| IBIS file generated by GenIBIS.pl Version 3.20
|   dm8168_pg2x
[IBIS ver]   4.1
[File name]   sprm568.ibs
[File Rev]   2.2
[Date]   Mon May 21, 2012, 13:39:56
[Source]   Data created at Texas Instruments
[Notes]   Checked with ibisckr
   16 warnings can be waived
   Some pins may contain selectors which are not valid options
   for that particular pin.
   Please refer to the device datasheet for information on picking
   the correct selector model, which depends on various software
   register configurations.
   Some pins are modeled as IO or tri-state for output mode.
[Disclaimer] Please be aware that in the absence of a written agreement,
   Texas Instruments (TI) assumes no liability for: 1) the
   accuracy of the IBIS models provided to your company, 2) the
   proper functioning of these IBIS models in your design or for
   any resulting applications, or, 3) infringement of patents,
   copyrights, or intellectual property rights resulting from
   your use of these IBIS models. TI provides IBIS models as a
   service to our customers and therefore reserves the right to
   limit distribution of the IBIS models.
[Copyright]   Property of Texas Instruments Incorporated. Unauthorised
   reproduction and/or distribution is strictly prohibited. This
   product is protected under copyright law and trade secret law
   as an unpublished work. Created 2010,(C) Copyright 2010,
   Texas Instruments Incorporated., All Rights Reserved. These
   commodities are under the U.S. Government distribution license
   control.As such,they are not to be re-exported without the
   prior approval of the U.S. Department of Commerce.
|   Component dm8168_pg2x
[Component]   dm8168_pg2x
[Manufacturer]   Texas Instruments.
| Source IO level model revisions
|Model   Revision   Date
|BSHTLTCSCDVGPBFZ   1.4   Jan 5, 2011
|IHHV33GP18   1.0   Feb 18, 2010
|BSHTLTCSCDDVGPBFZ   1.4   Jan 5, 2011
|BI2C33GFZP18   1.0   Feb 18, 2010
|BC3340CGHYPBFBP18   1.0   Feb 18, 2010
|BC3340DGHYPBFBP18   1.0   Feb 18, 2010
|IQ33GHYPBFBP18   1.0   Feb 18, 2010
[Package]
|   typ   min   max
R_pkg   1083.455m   49.41m   2117.50m
L_pkg   3.26nH   0.72nH   5.80nH
C_pkg   1.675pF   0.63pF   2.72pF
[Pin]   signal_name   model_name   R_pin   L_pin   C_pin
H37   CLKIN32   Selector_5   1309.20m   3.65nH   1.83pF
F1   CLKOUT   Selector_5   1491.00m   3.78nH   1.94pF
F18   DDR[0]_CS[1]N   Selector_6   1308.20m   3.34nH   1.73pF
G4   DDR[0]_D[3]   Selector_4   1490.40m   3.74nH   2.07pF
G34   DDR[1]_D[3]   Selector_4   1489.80m   3.78nH   2.08pF
C18   DDR[0]_CKE   Selector_6   1358.20m   3.54nH   1.63pF
N14   DDR[0]_A[8]   Selector_6   1151.50m   3.06nH   1.57pF
B2   DDR[0]_D[5]   Selector_4   1489.90m   3.72nH   2.04pF
A31   DDR[1]_D[17]   Selector_4   1477.60m   3.79nH   1.89pF
C29   DDR[1]_D[31]   Selector_4   1476.80m   3.76nH   1.94pF
F29   DDR[1]_D[22]   Selector_4   1441.70m   3.68nH   1.89pF
C37   DDR[1]_D[7]   Selector_4   1538.40m   3.97nH   2.11pF
D6   DDR[0]_D[11]   Selector_4   1736.00m   3.98nH   2.27pF
A7   DDR[0]_D[17]   Selector_4   1476.50m   3.78nH   1.93pF
J25   DDR[1]_A[5]   Selector_6   1309.60m   3.41nH   1.73pF
D32   DDR[1]_D[11]   Selector_4   1733.00m   4.16nH   2.21pF
B32   DDR[1]_D[13]   Selector_4   1708.80m   4.35nH   2.32pF
H25   DDR[1]_A[4]   Selector_6   1241.80m   3.15nH   1.69pF
B14   DDR[0]_BA[1]   Selector_6   1319.50m   3.63nH   1.86pF
C25   DDR[1]_CASN   Selector_6   1319.50m   3.60nH   1.85pF
B37   DDR[1]_D[0]   Selector_4   1469.70m   3.83nH   2.00pF
A32   DDR[1]_VTP   NC
B17   DDR[0]_CS[0]N   Selector_6   1349.40m   3.49nH   1.72pF
C8   DDR[0]_D[16]   Selector_4   1423.40m   3.34nH   1.91pF
A26   DDR[1]_CLK[0]N   Selector_6   1408.90m   3.58nH   1.67pF
B28   DDR[1]_D[26]   Selector_4   1457.10m   3.72nH   1.90pF
N21   DDR[1]_A[1]   Selector_6   1193.70m   3.19nH   1.60pF
B30   DDR[1]_DQS[2]   Selector_1   1543.40m   3.74nH   1.70pF
C14   DDR[0]_A[10]   Selector_6   1298.30m   3.51nH   1.79pF
F9   DDR[0]_D[22]   Selector_4   1439.50m   3.61nH   1.90pF
A9   DDR[0]_DQS[3]N   Selector_1   1585.40m   3.85nH   1.84pF
B7   DDR[0]_D[19]   Selector_4   1383.00m   3.34nH   1.95pF
A3   DDR[0]_D[14]   Selector_4   1766.10m   4.41nH   2.34pF
B1   DDR[0]_D[0]   Selector_4   1470.70m   3.76nH   2.13pF
A15   DDR[0]_CLK[1]   Selector_6   1409.10m   3.47nH   1.71pF
H13   DDR[0]_A[4]   Selector_6   1256.10m   3.18nH   1.74pF
D7   DDR[0]_D[9]   Selector_4   1744.10m   4.10nH   2.16pF
C24   DDR[1]_A[10]   Selector_6   1281.10m   3.40nH   1.81pF
D36   DDR[1]_D[4]   Selector_4   1532.20m   3.94nH   2.16pF
A35   DDR[1]_D[14]   Selector_4   1761.50m   4.48nH   2.31pF
F30   DDR[1]_D[20]   Selector_4   1426.70m   3.75nH   1.94pF
A4   DDR[0]_DQS[1]N   Selector_1   1881.10m   4.39nH   2.13pF
D31   DDR[1]_D[9]   Selector_4   1747.90m   4.19nH   2.19pF
A6   DDR[0]_VTP   NC
E18   DDR[0]_ODT[0]   Selector_6   1256.70m   3.57nH   1.67pF
B21   DDR[1]_CS[0]N   Selector_6   1338.00m   3.57nH   1.74pF
D20   DDR[1]_RSTN   Selector_6   1302.90m   3.49nH   1.67pF
N22   DDR[1]_A[12]   Selector_6   1129.60m   3.36nH   1.44pF
E2   DDR[0]_D[2]   Selector_4   1529.70m   3.83nH   2.00pF
A12   DDR[0]_CLK[0]N   Selector_6   1403.00m   3.48nH   1.71pF
G28   DDR[1]_D[28]   Selector_4   1477.50m   3.63nH   2.05pF
E29   DDR[1]_D[24]   NC
D30   DDR[1]_D[21]   Selector_4   1394.40m   3.59nH   1.98pF
C9   DDR[0]_D[31]   Selector_4   1469.70m   3.53nH   1.82pF
K13   DDR[0]_A[9]   Selector_6   1252.40m   3.22nH   1.70pF
G29   DDR[1]_DQM[2]   Selector_6   1449.00m   3.60nH   1.92pF
B3   DDR[0]_D[15]   Selector_4   1746.20m   4.07nH   2.26pF
A24   DDR[1]_A[7]   Selector_6   1317.50m   3.61nH   1.88pF
F36   DDR[1]_D[1]   Selector_4   1516.50m   3.72nH   2.10pF
B26   DDR[1]_CLK[0]   Selector_6   1421.50m   3.73nH   1.56pF
E7   DDR[0]_D[23]   NC
G13   DDR[0]_A[3]   Selector_6   1313.50m   3.47nH   1.69pF
B33   DDR[1]_DQM[1]   Selector_6   1739.30m   4.30nH   2.28pF
B35   DDR[1]_D[15]   Selector_4   1754.70m   4.28nH   2.24pF
G9   DDR[0]_DQM[2]   Selector_6   1448.90m   3.58nH   1.95pF
A30   DDR[1]_DQS[2]N   Selector_1   1544.90m   3.83nH   1.76pF
B10   DDR[0]_D[26]   Selector_4   1460.70m   3.63nH   1.97pF
E25   DDR[1]_WEN   Selector_6   1267.60m   3.39nH   1.80pF
F20   DDR[1]_CS[1]N   Selector_6   1298.80m   3.39nH   1.72pF
D18   DDR[0]_RSTN   Selector_6   1315.90m   3.41nH   1.71pF
F8   DDR[0]_D[20]   Selector_4   1427.80m   3.64nH   1.98pF
A34   DDR[1]_DQS[1]N   Selector_1   1885.10m   4.38nH   2.14pF
E36   DDR[1]_D[2]   Selector_4   1529.70m   3.92nH   2.08pF
A29   DDR[1]_DQS[3]N   Selector_1   1598.60m   3.83nH   1.94pF
G10   DDR[0]_D[28]   Selector_4   1486.50m   3.61nH   2.07pF
E35   DDR[1]_DQS[0]N   Selector_1   1600.60m   3.84nH   1.86pF
A13   DDR[0]_A[0]   Selector_6   1265.50m   3.65nH   1.74pF
E8   DDR[0]_D[27]   Selector_4   1430.00m   3.59nH   1.99pF
B9   DDR[0]_DQS[3]   Selector_1   1600.40m   3.82nH   1.84pF
F25   DDR[1]_BA[0]   Selector_6   1249.40m   3.21nH   1.71pF
E31   DDR[1]_D[23]   Selector_4   1404.30m   3.60nH   2.03pF
F13   DDR[0]_BA[0]   Selector_6   1260.70m   3.24nH   1.75pF
B11   DDR[0]_D[25]   Selector_4   1487.80m   3.56nH   1.92pF
J13   DDR[0]_A[5]   Selector_6   1333.50m   3.39nH   1.68pF
C13   DDR[0]_CASN   Selector_6   1332.10m   3.61nH   1.86pF
B25   DDR[1]_A[11]   Selector_6   1335.80m   3.85nH   1.84pF
J11   DDR[0]_D[30]   Selector_4   1504.00m   3.69nH   1.90pF
A8   DDR[0]_DQS[2]N   Selector_1   1538.30m   3.73nH   1.90pF
D8   DDR[0]_D[21]   Selector_4   1394.50m   3.33nH   2.05pF
A33   DDR[1]_D[12]   Selector_4   1736.90m   4.33nH   2.28pF
C11   DDR[0]_D[29]   Selector_4   1449.60m   3.76nH   1.97pF
A5   DDR[0]_D[12]   Selector_4   1740.90m   4.25nH   2.37pF
D15   DDR[0]_A[2]   Selector_6   1293.60m   3.44nH   1.80pF
B4   DDR[0]_DQS[1]   Selector_1   1878.40m   4.27nH   2.13pF
C30   DDR[1]_D[16]   Selector_4   1420.60m   3.50nH   2.00pF
B29   DDR[1]_DQS[3]   Selector_1   1607.10m   4.02nH   1.86pF
H10   DDR[0]_D[18]   Selector_4   1427.20m   3.35nH   2.06pF
E13   DDR[0]_WEN   Selector_6   1287.90m   3.35nH   1.78pF
D17   DDR[0]_A[14]   Selector_6   1253.70m   3.19nH   1.81pF
A25   DDR[1]_A[0]   Selector_6   1266.80m   3.73nH   1.79pF
C32   DDR[1]_D[10]   Selector_4   1784.80m   4.48nH   2.18pF
B13   DDR[0]_A[11]   Selector_6   1352.50m   3.67nH   1.95pF
A14   DDR[0]_A[7]   NC
F2   DDR[0]_D[1]   Selector_4   1518.50m   3.74nH   2.08pF
B36   DDR[1]_D[5]   Selector_4   1496.60m   3.79nH   2.09pF
L13   DDR[0]_A[6]   Selector_6   1153.10m   3.02nH   1.61pF
H28   DDR[1]_D[18]   Selector_4   1427.50m   3.48nH   1.90pF
F35   DDR[1]_D[6]   Selector_4   1543.90m   3.99nH   2.08pF
N16   DDR[0]_A[12]   Selector_6   1122.70m   3.13nH   1.44pF
B34   DDR[1]_DQS[1]   Selector_1   1881.40m   4.41nH   2.08pF
C36   DDR[1]_DQM[0]   Selector_6   1526.50m   4.01nH   2.09pF
F34   DDR[1]_DQS[0]   Selector_1   1622.30m   3.89nH   1.76pF
L25   DDR[1]_A[6]   Selector_6   1146.20m   2.92nH   1.59pF
A23   DDR[1]_CLK[1]   Selector_6   1408.60m   3.54nH   1.77pF
A22   DDR[1]_ODT[1]   Selector_6   1360.60m   3.61nH   1.87pF
F4   DDR[0]_DQS[0]   Selector_1   1620.50m   3.95nH   1.97pF
D25   DDR[1]_RASN   Selector_6   1251.90m   3.31nH   1.80pF
D21   DDR[1]_A[14]   Selector_6   1262.30m   3.15nH   1.77pF
D29   DDR[1]_DQM[3]   Selector_6   1482.20m   3.81nH   2.01pF
B16   DDR[0]_A[13]   Selector_6   1270.10m   3.37nH   1.81pF
N15   DDR[0]_BA[2]   Selector_6   1133.30m   3.22nH   1.44pF
E30   DDR[1]_D[27]   Selector_4   1425.40m   3.68nH   2.08pF
B27   DDR[1]_D[25]   Selector_4   1494.60m   3.90nH   1.92pF
C20   DDR[1]_CKE   Selector_6   1327.50m   3.43nH   1.63pF
N24   DDR[1]_A[8]   Selector_6   1151.30m   3.03nH   1.54pF
B12   DDR[0]_CLK[0]   Selector_6   1415.20m   3.69nH   1.69pF
B6   DDR[0]_D[13]   Selector_4   1710.40m   4.12nH   2.18pF
N23   DDR[1]_BA[2]   Selector_6   1141.30m   3.31nH   1.43pF
F3   DDR[0]_D[6]   Selector_4   1543.60m   4.02nH   2.09pF
C27   DDR[1]_D[29]   Selector_4   1448.30m   3.80nH   2.01pF
E9   DDR[0]_D[24]   Selector_4   1434.50m   3.63nH   1.86pF
J27   DDR[1]_D[30]   Selector_4   1507.60m   3.72nH   2.06pF
E20   DDR[1]_ODT[0]   Selector_6   1246.60m   3.51nH   1.69pF
B24   DDR[1]_BA[1]   Selector_6   1300.70m   3.55nH   1.82pF
A16   DDR[0]_ODT[1]   Selector_6   1375.80m   3.74nH   1.86pF
D13   DDR[0]_RASN   Selector_6   1266.70m   3.18nH   1.82pF
D2   DDR[0]_D[4]   Selector_4   1531.00m   3.98nH   2.12pF
D23   DDR[1]_A[2]   Selector_6   1279.00m   3.38nH   1.87pF
D9   DDR[0]_DQM[3]   Selector_6   1479.60m   3.74nH   1.92pF
B15   DDR[0]_CLK[1]N   Selector_6   1400.90m   3.42nH   1.71pF
N17   DDR[0]_A[1]   Selector_6   1196.40m   3.20nH   1.58pF
G25   DDR[1]_A[3]   Selector_6   1301.50m   3.47nH   1.74pF
K25   DDR[1]_A[9]   Selector_6   1252.70m   3.22nH   1.71pF
B31   DDR[1]_D[19]   Selector_4   1383.90m   3.59nH   1.84pF
E3   DDR[0]_DQS[0]N   Selector_1   1601.30m   3.84nH   1.94pF
B5   DDR[0]_DQM[1]   Selector_6   1739.40m   4.39nH   2.24pF
C33   DDR[1]_D[8]   NC
B22   DDR[1]_A[13]   Selector_6   1250.70m   3.43nH   1.78pF
B8   DDR[0]_DQS[2]   Selector_1   1535.10m   3.81nH   1.76pF
C5   DDR[0]_D[8]   Selector_4   1688.70m   3.78nH   2.09pF
B23   DDR[1]_CLK[1]N   Selector_6   1400.10m   3.58nH   1.69pF
C6   DDR[0]_D[10]   Selector_4   1782.00m   4.37nH   2.22pF
C2   DDR[0]_DQM[0]   Selector_6   1527.40m   3.89nH   2.14pF
C1   DDR[0]_D[7]   NC
A19   DEV_MXI   NC
C19   DEV_MXO   NC
AU31   EMAC[1]_TXD[4]   Selector_2   1696.40m   4.60nH   2.24pF
AD35   EMAC[0]_RXD[3]   Selector_2   947.25m   2.61nH   1.46pF
AT31   EMAC[1]_TXD[5]   Selector_2   1489.10m   4.26nH   1.93pF
AU30   EMAC[1]_TXEN   Selector_2   1493.30m   4.07nH   2.01pF
AU36   EMAC[1]_RXD[2]   Selector_2   1943.20m   4.97nH   2.40pF
AE36   EMAC[0]_RXD[7]   Selector_2   1288.30m   3.53nH   1.68pF
AU33   EMAC[1]_GMTCLK   Selector_2   1708.70m   4.59nH   2.17pF
AG36   EMAC[0]_TXD[6]   Selector_2   1331.80m   3.61nH   1.78pF
AT37   EMAC[1]_RXCLK   Selector_2   1743.20m   4.77nH   2.32pF
AT35   EMAC[1]_RXD[1]   Selector_2   1674.40m   4.57nH   2.13pF
AB25   EMAC[0]_COL   Selector_2   226.60m   1.06nH   0.71pF
AF37   EMAC[0]_TXCLK   Selector_2   1350.00m   3.67nH   1.87pF
AG37   EMAC[0]_TXEN   Selector_2   1452.10m   3.88nH   1.95pF
AT34   EMAC[1]_RXD[3]   Selector_2   1793.70m   4.65nH   2.21pF
AG35   EMAC[0]_TXD[7]   Selector_2   1051.50m   2.91nH   1.59pF
AT30   EMAC[1]_TXCLK   Selector_2   1568.10m   4.28nH   2.08pF
AE37   EMAC[0]_RXCLK   Selector_2   1509.90m   3.89nH   2.04pF
AD25   EMAC[0]_RXD[5]   Selector_2   170.60m   1.01nH   0.78pF
AC35   EMAC[0]_RXD[4]   Selector_2   1124.40m   3.09nH   1.69pF
AR33   EMAC[1]_RXD[5]   Selector_2   1589.90m   4.08nH   2.09pF
AP30   EMAC[1]_TXD[6]   Selector_2   1528.60m   4.24nH   1.97pF
AF36   EMAC[0]_TXD[5]   Selector_2   1240.00m   3.21nH   1.63pF
AP31   EMAC[1]_TXD[0]   Selector_2   1401.40m   3.88nH   1.91pF
AU32   EMAC[1]_TXD[3]   Selector_2   1538.00m   4.30nH   2.17pF
AE35   EMAC[0]_RXDV   Selector_2   1056.10m   2.91nH   1.55pF
AC36   EMAC[0]_RXD[2]   Selector_2   1200.10m   3.19nH   1.70pF
AP32   EMAC[1]_RXD[7]   Selector_2   1347.40m   3.62nH   1.88pF
AR32   EMAC[1]_TXD[1]   Selector_2   1395.10m   3.95nH   1.95pF
AE32   EMAC[0]_TXD[1]   Selector_2   762.14m   2.22nH   1.20pF
AU35   EMAC[1]_RXD[4]   Selector_2   1865.90m   4.74nH   2.42pF
AG28   EMAC[0]_TXD[4]   Selector_2   564.85m   1.69nH   1.08pF
AD37   EMAC[0]_RXD[0]   Selector_2   1306.50m   3.47nH   1.77pF
AD36   EMAC[0]_RXD[1]   Selector_2   1427.60m   3.90nH   1.76pF
AN30   EMAC[1]_RXER   Selector_2   1352.10m   3.58nH   1.79pF
AE31   EMAC[0]_TXD[2]   Selector_2   828.93m   2.29nH   1.22pF
AC25   EMAC[0]_RXD[6]   Selector_2   92.81m   0.81nH   0.65pF
AC37   EMAC[0]_GMTCLK   Selector_2   1221.60m   3.13nH   1.69pF
AR30   EMAC[1]_COL   Selector_2   1353.40m   3.90nH   1.89pF
AE33   EMAC[0]_TXD[0]   Selector_2   986.48m   2.66nH   1.40pF
AN31   EMAC[1]_CRS   Selector_2   1339.00m   3.72nH   1.83pF
AT32   EMAC[1]_TXD[2]   Selector_2   1667.80m   4.59nH   2.05pF
AE30   EMAC[0]_TXD[3]   Selector_2   493.69m   1.61nH   1.01pF
AU34   EMAC[1]_RXD[6]   Selector_2   1858.20m   5.09nH   2.51pF
AT36   EMAC[1]_RXD[0]   Selector_2   1623.80m   4.40nH   2.14pF
AE34   EMAC[0]_RXER   Selector_2   916.91m   2.56nH   1.42pF
AM30   EMAC[1]_TXD[7]   Selector_2   1204.30m   3.33nH   1.65pF
AA25   EMAC[0]_CRS   Selector_2   100.59m   0.85nH   0.71pF
AT33   EMAC[1]_RXDV   Selector_2   1519.30m   4.11nH   2.10pF
J35   EMU0   Selector_2   1645.80m   4.47nH   2.22pF
L36   EMU1   Selector_2   1287.90m   3.82nH   1.76pF
L37   EMU2   Selector_2   1334.20m   3.65nH   1.85pF
M36   EMU3   Selector_2   1079.80m   3.03nH   1.65pF
M37   EMU4   Selector_2   1302.60m   3.45nH   1.77pF
K31   GP0[0]   Selector_5   795.97m   2.24nH   1.35pF
L29   GP0[1]   Selector_5   694.30m   2.11nH   1.26pF
G2   GP0[5]   Selector_5   1205.80m   3.58nH   1.79pF
H35   GP0[7]   Selector_5   1083.40m   3.13nH   1.75pF
H32   GP0[4]   Selector_5   1092.10m   2.82nH   1.67pF
G5   GP0[6]   Selector_5   1196.30m   3.27nH   1.74pF
J31   GP0[3]   Selector_5   1017.90m   2.83nH   1.55pF
H4   GP0[25]   Selector_5   1249.30m   3.40nH   1.66pF
AC5   GP0[20]   Selector_5   1270.00m   3.50nH   1.93pF
K30   GP0[2]   Selector_5   925.22m   2.65nH   1.41pF
J5   GP1[13]   Selector_5   1061.30m   3.17nH   1.63pF
J32   GP1[30]   Selector_5   1020.50m   2.79nH   1.56pF
J33   GP1[31]   Selector_5   1137.80m   3.33nH   1.68pF
AA2   GPMC_D[5]   Selector_5   1118.40m   3.28nH   1.58pF
AE2   GPMC_A[5]   Selector_5   1495.60m   3.99nH   1.96pF
AE1   GPMC_A[4]   Selector_5   1377.50m   3.92nH   1.90pF
J1   GPMC_A[15]   Selector_5   1395.10m   3.87nH   1.92pF
AH7   GPMC_CS[0]N   Selector_5   1189.60m   3.37nH   1.71pF
AE6   GPMC_A[0]   Selector_5   1350.00m   3.73nH   2.00pF
AG9   GPMC_CS[3]N   Selector_5   1366.30m   3.85nH   2.05pF
AA3   GPMC_D[3]   Selector_5   1056.40m   2.99nH   1.56pF
W1   GPMC_D[11]   Selector_5   1141.60m   3.23nH   1.64pF
Y2   GPMC_D[7]   Selector_5   1171.80m   3.24nH   1.63pF
W2   GPMC_D[12]   Selector_5   966.20m   2.79nH   1.53pF
J2   GPMC_A[16]   Selector_5   1182.70m   3.29nH   1.76pF
Y1   GPMC_D[9]   Selector_5   1157.00m   3.26nH   1.75pF
AB2   GPMC_D[2]   Selector_5   1290.40m   3.51nH   1.73pF
AG2   GPMC_WEN   Selector_5   1545.10m   4.10nH   2.08pF
V3   GPMC_D[14]   Selector_5   1008.30m   2.79nH   1.47pF
W3   GPMC_D[10]   Selector_5   1112.50m   3.04nH   1.53pF
Y10   GPMC_D[6]   Selector_5   352.48m   1.25nH   0.89pF
AE3   GPMC_A[3]   Selector_5   1358.60m   3.79nH   1.85pF
V10   GPMC_D[13]   Selector_5   184.75m   0.89nH   0.73pF
AC1   GPMC_D[0]   Selector_5   1233.50m   3.39nH   1.85pF
V1   GPMC_CLK   Selector_5   1272.40m   3.48nH   1.79pF
K8   GPMC_A[27]   Selector_5   879.20m   2.55nH   1.43pF
J3   GPMC_A[24]   Selector_5   1308.40m   3.54nH   1.75pF
K2   GPMC_A[22]   Selector_5   1115.70m   3.16nH   1.71pF
AD8   GPMC_A[6]   Selector_5   1530.30m   4.11nH   2.05pF
AC2   GPMC_A[11]   Selector_5   1362.40m   3.66nH   1.85pF
AE4   GPMC_A[2]   Selector_5   1235.40m   3.43nH   1.67pF
AH2   GPMC_CS[2]N   Selector_5   1411.50m   3.83nH   2.11pF
AD3   GPMC_A[7]   Selector_5   1196.70m   3.32nH   1.73pF
Y3   GPMC_D[4]   Selector_5   1143.00m   3.16nH   1.62pF
J6   GPMC_A[26]   Selector_5   1225.70m   3.47nH   1.74pF
AD4   GPMC_A[8]   Selector_5   1152.80m   3.26nH   1.73pF
H5   GPMC_A[14]   Selector_5   1173.60m   3.57nH   1.70pF
AD1   GPMC_A[10]   Selector_5   1395.90m   3.72nH   1.87pF
W4   GPMC_D[8]   Selector_5   980.65m   2.85nH   1.47pF
AE7   GPMC_DIR   Selector_5   1320.10m   3.72nH   1.87pF
H3   GPMC_A[21]   Selector_5   1193.00m   3.32nH   1.78pF
AE10   GPMC_ADVN_ALE   Selector_5   1720.10m   4.77nH   2.21pF
AD2   GPMC_A[9]   Selector_5   1429.00m   3.83nH   1.94pF
H2   GPMC_A[12]   Selector_5   1117.60m   3.22nH   1.57pF
J4   GPMC_A[23]   Selector_5   1051.60m   2.94nH   1.64pF
H6   GPMC_A[13]   Selector_5   1045.70m   3.38nH   1.56pF
AE11   GPMC_BE0N_CLE   Selector_5   532.49m   1.84nH   1.17pF
AE9   GPMC_WPN   Selector_5   1318.70m   3.47nH   1.88pF
AH1   GPMC_CS[1]N   Selector_5   1653.70m   4.70nH   2.01pF
AF1   GPMC_BE1N   Selector_5   1416.40m   3.85nH   2.00pF
AE8   GPMC_WAIT   Selector_5   1441.30m   4.00nH   1.90pF
J7   GPMC_A[25]   Selector_5   1173.20m   3.20nH   1.70pF
AE5   GPMC_A[1]   Selector_5   1097.80m   3.10nH   1.66pF
AF2   GPMC_OE_REN   Selector_5   1476.20m   3.88nH   1.94pF
V2   GPMC_D[15]   Selector_5   1141.50m   3.10nH   1.63pF
AA4   GPMC_D[1]   Selector_5   1051.20m   2.95nH   1.51pF
AG3   GPMC_CS[4]N   Selector_5   1297.50m   3.69nH   1.80pF
AG1   GPMC_CS[5]N   Selector_5   1663.40m   4.38nH   2.09pF
AE24   HDMI_HPDET   Selector_5   316.48m   1.39nH   0.87pF
AT26   HDMI_TMDSDP1   NC
AT25   HDMI_TMDSDP0   NC
AU24   HDMI_TMDSCLKN   NC
AP25   HDMI_CEC   Selector_5   1161.80m   3.19nH   1.63pF
AU25   HDMI_TMDSDN0   NC
AU26   HDMI_TMDSDN1   NC
AL25   HDMI_SCL   Model_275   1122.30m   3.12nH   1.65pF
AN25   HDMI_EXTSWING   NC
AT27   HDMI_TMDSDP2   NC
AT24   HDMI_TMDSCLKP   NC
AK25   HDMI_SDA   Model_275   1029.40m   2.70nH   1.63pF
AU27   HDMI_TMDSDN2   NC
N34   I2C[1]_SCL   Model_275   975.35m   2.79nH   1.48pF
N32   I2C[0]_SCL   Model_275   612.69m   1.99nH   1.17pF
N35   I2C[1]_SDA   Model_275   1136.40m   3.15nH   1.69pF
N33   I2C[0]_SDA   Model_275   750.94m   2.35nH   1.20pF
AT21   IOUTA   NC
AR21   IOUTB   NC
AP21   IOUTC   NC
AR20   IOUTD   NC
AT19   IOUTE   NC
AT20   IOUTF   NC
AU20   IOUTG   NC
AK37   MCA[0]_AXR[0]   Selector_5   1454.10m   3.84nH   1.91pF
AM37   MCA[1]_AHCLKX   Selector_5   1557.70m   4.14nH   2.05pF
AJ37   MCA[0]_AXR[5]   Selector_5   1303.30m   3.38nH   1.90pF
AJ35   MCA[0]_AMUTE   Selector_5   1238.10m   3.28nH   1.65pF
AL33   MCA[1]_AXR[0]   Selector_5   1175.20m   3.24nH   1.75pF
AN36   MCA[2]_AHCLKX   Selector_5   1652.90m   4.24nH   2.15pF
AK28   MCA[0]_ACLKR   Selector_5   691.13m   2.17nH   1.19pF
AR37   MCA[2]_AXR[1]   Selector_5   1784.60m   4.90nH   2.34pF
AL37   MCA[1]_AHCLKR   Selector_5   1549.50m   4.00nH   2.09pF
AJ32   MCA[0]_AXR[1]   Selector_5   1267.10m   3.43nH   1.71pF
AJ31   MCA[0]_AFSX   Selector_5   946.20m   2.58nH   1.39pF
AR36   MCA[2]_AXR[0]   Selector_5   1739.00m   4.42nH   2.24pF
AM36   MCA[2]_ACLKX   Selector_5   1446.70m   4.09nH   1.93pF
AP36   MCA[2]_AMUTE   Selector_5   1538.80m   4.58nH   2.10pF
AM35   MCA[2]_AFSR   Selector_5   1487.90m   4.07nH   1.90pF
AL34   MCA[2]_ACLKR   Selector_5   1200.30m   3.13nH   1.75pF
AK32   MCA[1]_AXR[1]   Selector_5   1015.70m   2.72nH   1.48pF
AK35   MCA[1]_AFSR   Selector_5   1404.40m   3.71nH   2.00pF
AK36   MCA[1]_ACLKR   Selector_5   1296.00m   3.73nH   1.90pF
AL36   MCA[1]_ACLKX   Selector_5   1648.10m   4.37nH   2.19pF
AJ27   MCA[0]_AHCLKR   Selector_5   528.21m   1.54nH   1.02pF
AH30   MCA[0]_ACLKX   Selector_5   727.97m   2.17nH   1.16pF
AN35   MCA[2]_AFSX   Selector_5   1404.00m   3.87nH   2.02pF
AJ34   MCA[0]_AXR[3]   Selector_5   1356.50m   3.64nH   1.82pF
AK34   MCA[1]_AFSX   Selector_5   1182.80m   3.36nH   1.76pF
AH31   MCA[0]_AHCLKX   Selector_5   808.09m   2.43nH   1.29pF
AG29   MCA[0]_AFSR   Selector_5   574.77m   1.74nH   1.06pF
AJ33   MCA[0]_AXR[2]   Selector_5   1310.90m   3.50nH   1.79pF
AJ36   MCA[0]_AXR[4]   Selector_5   1321.90m   3.59nH   1.93pF
AM34   MCA[2]_AHCLKR   Selector_5   1381.00m   3.66nH   1.84pF
AK33   MCA[1]_AMUTE   Selector_5   1127.60m   2.94nH   1.66pF
AH36   MDIO_MDIO   Selector_5   1172.50m   3.05nH   1.63pF
AH37   MDIO_MCLK   Selector_5   1273.70m   3.46nH   1.85pF
G36   NMIN   Selector_5   1218.30m   3.39nH   1.76pF
Y27   PCIE_TXP1   NC
AB31   PCIE_TXP0   NC
V29   PCIE_RXN0   NC
V31   PCIE_RXP1   NC
Y29   PCIE_RXP0   NC
AB28   PCIE_TXN1   NC
AB30   PCIE_TXN0   NC
V30   PCIE_RXN1   NC
F37   PORN   Model_1   1487.00m   3.97nH   1.84pF
G33   RESETN   Selector_5   1164.50m   3.18nH   1.65pF
G37   RSTOUTN   Selector_5   1491.30m   4.03nH   2.05pF
AB36   RSV1   NC
P25   RSV2   NC
N19   RSV3   NC
N20   RSV4   NC
T28   RSV5   NC
T27   RSV6   NC
AE23   RSV7   NC
AU37   RSV9   NC
N28   RSV10   NC
N29   RSV11   NC
R34   RSV16   NC
P34   RSV17   NC
AP2   RSV23   Selector_2   1694.20m   4.68nH   2.23pF
AU3   RSV24   Selector_2   2117.50m   5.77nH   2.72pF
AN2   RSV25   Selector_2   1543.30m   4.17nH   2.20pF
AT1   RSV26   Selector_2   1979.70m   5.80nH   2.46pF
AR1   RSV27   Selector_2   1802.10m   5.00nH   2.40pF
AP1   RSV28   Selector_2   1650.20m   4.42nH   2.28pF
AM2   RSV29   Selector_2   1471.90m   4.29nH   2.02pF
AL2   RSV30   Selector_2   1458.20m   4.17nH   2.00pF
AK1   RSV31   Selector_2   1622.70m   4.67nH   2.10pF
AL1   RSV32   Selector_2   1673.30m   4.64nH   2.18pF
AM29   RSV33   Selector_5   1260.30m   3.63nH   1.76pF
AL28   RSV34   Selector_5   999.58m   2.85nH   1.59pF
AL29   RSV35   Selector_5   1165.90m   3.32nH   1.56pF
AN29   RSV36   Selector_5   1177.60m   3.06nH   1.62pF
AP29   RSV37   Selector_5   1198.90m   3.48nH   1.75pF
AR29   RSV38   Selector_5   1416.30m   3.63nH   1.90pF
AT29   RSV39   Selector_5   1429.70m   4.08nH   1.87pF
AT28   RSV40   Selector_5   1200.10m   3.31nH   1.74pF
AU21   RSV41   NC
AJ1   RSV42   Selector_2   1624.10m   4.48nH   2.15pF
AK2   RSV43   Selector_2   1410.60m   3.93nH   1.94pF
AH8   RSV44   Selector_2   1099.90m   3.07nH   1.58pF
AJ2   RSV45   Selector_2   1514.70m   4.21nH   2.05pF
AK3   RSV46   Selector_2   1529.30m   4.11nH   2.10pF
AJ3   RSV47   Selector_2   1462.40m   4.01nH   1.99pF
AJ4   RSV48   Selector_2   1241.90m   3.63nH   1.87pF
AJ5   RSV49   Selector_2   1264.90m   3.50nH   1.90pF
AJ6   RSV50   Selector_2   1343.60m   3.71nH   1.89pF
AB13   RSV51   Selector_2   160.17m   0.98nH   0.78pF
J36   RTCK   Selector_5   1441.60m   3.91nH   1.92pF
T31   SATA_TXN0   NC
U33   SATA_TXN1   NC
V36   SATA_RXP0   NC
T32   SATA_TXP0   NC
V37   SATA_RXN0   NC
V35   SATA_RXN1   NC
W35   SATA_RXP1   NC
V33   SATA_TXP1   NC
T13   SD_DAT[3]   Selector_5   271.80m   1.19nH   0.84pF
T2   SD_DAT[2]_SDRW   Selector_5   1149.00m   3.23nH   1.66pF
U1   SD_DAT[0]   Selector_5   1206.20m   3.39nH   1.68pF
U4   SD_POW   Selector_5   829.64m   2.47nH   1.30pF
R13   SD_SDCD   Selector_5   221.26m   1.25nH   0.82pF
R5   SD_SDWP   Selector_5   904.81m   2.64nH   1.32pF
U3   SD_CMD   Selector_5   992.29m   2.99nH   1.45pF
T1   SD_DAT[1]_SDIRQ   Selector_5   1078.00m   3.08nH   1.60pF
U2   SD_CLK   Selector_5   975.81m   2.83nH   1.48pF
AB34   SERDES_CLKP   NC
AB33   SERDES_CLKN   NC
P1   SPI_SCS[3]N   Selector_5   1096.00m   3.15nH   1.70pF
P3   SPI_SCS[2]N   Selector_5   987.83m   2.80nH   1.53pF
P13   SPI_D[1]   Selector_5   145.99m   0.87nH   0.73pF
P2   SPI_SCS[1]N   Selector_5   1213.40m   3.45nH   1.69pF
R2   SPI_SCLK   Selector_5   1165.00m   3.30nH   1.69pF
R1   SPI_SCS[0]N   Selector_5   1135.00m   3.30nH   1.57pF
N11   SPI_D[0]   Selector_5   510.79m   1.68nH   1.05pF
J37   TCLK   Selector_3   1317.20m   3.79nH   1.87pF
J34   TDI   Selector_3   1591.40m   4.51nH   2.12pF
N30   TDO   Selector_2   623.22m   1.99nH   1.23pF
H33   TIM4_OUT   Selector_5   1137.00m   3.34nH   1.66pF
H34   TIM5_OUT   Selector_5   1275.80m   3.46nH   1.79pF
H1   TIM6_OUT   Selector_5   1253.50m   3.62nH   1.76pF
G1   TIM7_OUT   Selector_5   1398.80m   4.13nH   1.83pF
N31   TMS   Selector_5   700.89m   2.16nH   1.32pF
K36   TRSTN   Selector_3   1293.50m   3.74nH   1.76pF
N8   UART0_TXD   Selector_5   868.60m   2.50nH   1.32pF
N10   UART0_RXD   Selector_5   748.15m   2.28nH   1.19pF
N9   UART0_RTSN   Selector_5   628.93m   1.93nH   1.12pF
N6   UART0_DTRN   Selector_5   922.02m   2.79nH   1.39pF
N5   UART0_DCDN   Selector_5   827.57m   2.44nH   1.40pF
N7   UART0_CTSN   Selector_5   705.88m   2.28nH   1.24pF
N4   UART0_DSRN   Selector_5   994.06m   2.84nH   1.50pF
N3   UART0_RIN   Selector_5   1130.30m   3.18nH   1.60pF
L3   UART1_CTSN   Selector_5   1169.80m   3.36nH   1.60pF
M2   UART1_RTSN   Selector_5   1056.30m   3.10nH   1.76pF
N2   UART1_TXD   Selector_5   1125.70m   3.22nH   1.54pF
N1   UART1_RXD   Selector_5   1089.60m   3.17nH   1.69pF
K7   UART2_CTSN   Selector_5   945.39m   2.78nH   1.51pF
M1   UART2_RXD   Selector_5   1382.50m   3.76nH   1.92pF
L2   UART2_TXD   Selector_5   1115.30m   3.17nH   1.66pF
L9   UART2_RTSN   Selector_5   842.24m   2.44nH   1.23pF
N37   USB0_R1   NC
P35   USB0_DRVVBUS   Model_274   1089.00m   3.00nH   1.60pF
P36   USB0_DN   NC
P37   USB0_DP   NC
R36   USB1_DN   NC
T37   USB1_R1   NC
R35   USB1_DRVVBUS   Model_274   979.53m   2.82nH   1.54pF
R37   USB1_DP   NC
AH19   VDAC_VREF   NC
N36   VDD_USB0_VBUS   NC
T36   VDD_USB1_VBUS   NC
AU15   VIN[0]A_D[14]   Selector_2   1374.00m   3.75nH   1.78pF
AR18   VIN[0]A_D[3]   Selector_2   1492.40m   4.06nH   1.92pF
AL5   VIN[0]A_D[17]   Selector_2   1078.00m   3.24nH   1.61pF
AN3   VIN[0]A_D[20]   Selector_2   1465.70m   4.13nH   2.11pF
AU14   VIN[0]A_D[15]   Selector_2   1352.60m   3.58nH   1.84pF
AH18   VIN[0]A_D[2]   Selector_2   872.75m   2.31nH   1.32pF
AT2   VIN[0]A_D[23]   Selector_2   1749.50m   4.88nH   2.30pF
AE16   VIN[0]A_D[9]   Selector_2   131.92m   0.96nH   0.74pF
AT15   VIN[0]A_D[13]   Selector_2   1198.30m   3.34nH   1.74pF
AL4   VIN[0]A_FLD   Selector_2   1190.50m   3.43nH   1.71pF
AP18   VIN[0]A_D[6]   Selector_2   1420.70m   3.57nH   1.86pF
AU5   VIN[0]A_HSYNC   Selector_2   1870.90m   4.92nH   2.39pF
AR14   VIN[0]A_CLK   Selector_2   1177.50m   3.33nH   1.81pF
AT18   VIN[0]A_D[4]   Selector_2   1510.80m   4.01nH   1.96pF
AR2   VIN[0]A_D[22]   Selector_2   1623.10m   4.50nH   2.18pF
AR17   VIN[0]A_D[7]   Selector_2   1254.10m   3.52nH   1.68pF
AU16   VIN[0]A_D[12]   Selector_2   1315.80m   3.94nH   1.86pF
AT17   VIN[0]A_D[5]   Selector_2   1241.40m   3.52nH   1.84pF
AU4   VIN[0]A_D[21]   Selector_2   2068.40m   5.19nH   2.61pF
AP17   VIN[0]A_D[8]   Selector_2   1257.20m   3.41nH   1.78pF
AK4   VIN[0]A_D[19]   Selector_2   1433.00m   4.30nH   2.02pF
AM3   VIN[1]A_D[14]   Selector_2   1486.90m   4.13nH   2.13pF
AR19   VIN[0]B_CLK   Selector_2   1341.60m   3.64nH   1.82pF
AT3   VIN[0]A_DE   Selector_2   1774.10m   4.84nH   2.32pF
AK5   VIN[0]A_D[18]   Selector_2   1069.10m   3.00nH   1.67pF
AU17   VIN[0]A_D[11]   Selector_2   1491.10m   4.08nH   1.87pF
AU18   VIN[0]A_D[1]   Selector_2   1358.60m   3.72nH   1.93pF
AT5   VIN[0]A_D[16]   Selector_2   1629.60m   4.24nH   2.16pF
AJ19   VIN[0]A_D[0]   Selector_2   1023.40m   2.63nH   1.45pF
AM4   VIN[0]A_VSYNC   Selector_2   1322.30m   3.61nH   1.91pF
AT16   VIN[0]A_D[10]   Selector_2   1230.30m   3.72nH   1.71pF
AJ13   VOUT[0]_B_CB_C[6]   Selector_2   548.25m   1.76nH   1.05pF
AT4   VOUT[1]_AVID   Selector_2   1755.50m   4.94nH   2.26pF
AN9   VOUT[0]_VSYNC   Selector_2   1032.00m   2.99nH   1.55pF
AD13   VOUT[1]_C[7]   Selector_2   104.10m   0.86nH   0.69pF
AR13   VOUT[0]_G_Y_YC[9]   Selector_2   1023.70m   2.96nH   1.49pF
AP8   VOUT[1]_C[5]   Selector_2   1276.80m   3.77nH   1.72pF
AU10   VOUT[0]_R_CR[6]   Selector_2   1382.50m   3.58nH   1.80pF
AL14   VOUT[0]_G_Y_YC[4]   Selector_2   1234.60m   3.55nH   1.77pF
AT9   VOUT[0]_B_CB_C[1]   Selector_2   1193.10m   3.31nH   1.65pF
AN13   VOUT[0]_B_CB_C[4]   Selector_2   863.96m   2.52nH   1.28pF
AU6   VOUT[1]_Y_YC[4]   Selector_2   1546.80m   4.48nH   2.10pF
AP14   VOUT[0]_G_Y_YC[3]   Selector_2   1087.90m   2.97nH   1.55pF
AP7   VOUT[1]_Y_YC[3]   Selector_2   1378.80m   3.95nH   1.76pF
AG13   VOUT[0]_R_CR[4]   Selector_2   217.78m   1.00nH   0.73pF
AK10   VOUT[0]_R_CR[8]   Selector_2   781.57m   2.22nH   1.14pF
AT6   VOUT[1]_Y_YC[8]   Selector_2   1571.00m   4.35nH   2.16pF
AK13   VOUT[0]_B_CB_C[5]   Selector_2   665.88m   2.05nH   1.13pF
AP9   VOUT[0]_G_Y_YC[0]   Selector_2   1029.30m   3.03nH   1.48pF
AK6   VOUT[1]_C[2]   Selector_2   988.10m   2.94nH   1.48pF
AP13   VOUT[0]_B_CB_C[2]   Selector_2   917.76m   2.65nH   1.36pF
AE15   VOUT[0]_G_Y_YC[2]   Selector_2   151.06m   0.89nH   0.76pF
AR9   VOUT[0]_B_CB_C[0]   Selector_2   1366.30m   3.49nH   1.73pF
AM9   VOUT[0]_HSYNC   Selector_2   1053.70m   2.93nH   1.49pF
AT8   VOUT[0]_R_CR[1]   Selector_2   1280.60m   3.58nH   1.81pF
AN8   VOUT[1]_C[6]   Selector_2   1361.20m   3.75nH   1.84pF
AM8   VOUT[1]_C[3]   Selector_2   955.08m   2.77nH   1.46pF
AT13   VOUT[0]_G_Y_YC[7]   Selector_2   1050.90m   3.01nH   1.60pF
AU8   VOUT[0]_G_Y_YC[1]   Selector_2   1507.00m   3.98nH   1.89pF
AN7   VOUT[1]_C[4]   Selector_2   1213.20m   3.57nH   1.77pF
AH13   VOUT[0]_B_CB_C[8]   Selector_2   489.34m   1.53nH   0.94pF
AM14   VOUT[0]_G_Y_YC[5]   Selector_2   968.59m   2.74nH   1.44pF
AT10   VOUT[0]_R_CR[5]   Selector_2   1370.10m   3.64nH   1.73pF
AR6   VOUT[1]_Y_YC[7]   Selector_2   1381.20m   3.80nH   1.90pF
AU9   VOUT[0]_R_CR[9]   Selector_2   1537.60m   3.98nH   1.92pF
AJ11   VOUT[0]_R_CR[0]   Selector_2   549.21m   1.80nH   1.00pF
AC13   VOUT[1]_Y_YC[6]   Selector_2   155.01m   1.03nH   0.72pF
AT7   VOUT[1]_CLK   Selector_2   1406.70m   3.83nH   2.00pF
AL10   VOUT[0]_R_CR[7]   Selector_2   789.95m   2.20nH   1.14pF
AT12   VOUT[0]_B_CB_C[9]   Selector_2   1085.10m   2.92nH   1.62pF
AT11   VOUT[0]_R_CR[2]   Selector_2   1157.90m   3.04nH   1.60pF
AU7   VOUT[1]_Y_YC[2]   Selector_2   1606.70m   4.46nH   2.06pF
AU13   VOUT[0]_G_Y_YC[8]   Selector_2   1388.60m   4.10nH   1.72pF
AP6   VOUT[1]_Y_YC[9]   Selector_2   1445.20m   4.18nH   1.89pF
AL13   VOUT[0]_B_CB_C[3]   Selector_2   690.20m   2.13nH   1.17pF
AL9   VOUT[0]_FLD   Selector_2   961.15m   2.67nH   1.40pF
AJ7   VOUT[1]_Y_YC[5]   Selector_2   1044.50m   3.12nH   1.54pF
AR5   VOUT[1]_HSYNC   Selector_2   1614.20m   4.48nH   2.10pF
AR11   VOUT[0]_R_CR[3]   Selector_2   1204.20m   3.21nH   1.49pF
AR8   VOUT[0]_AVID   Selector_2   1291.70m   3.62nH   1.76pF
AT14   VOUT[0]_CLK   Selector_2   1310.60m   3.66nH   1.77pF
AM13   VOUT[0]_B_CB_C[7]   Selector_2   856.98m   2.52nH   1.28pF
AE14   VOUT[0]_G_Y_YC[6]   Selector_2   49.41m   0.72nH   0.63pF
H36   WD_OUT   Selector_5   1132.30m   3.29nH   1.67pF
[Diff Pin]   inv_pin   vdiff   tdelay_typ
|DDR[1]_DQS[3]N   DDR[1]_DQS[3]
A29   B29   200m   NA
|DDR[0]_DQS[2]   DDR[0]_DQS[2]N
B8   A8   200m   NA
|DDR[0]_DQS[1]N   DDR[0]_DQS[1]
A4   B4   200m   NA
|DDR[0]_DQS[3]N   DDR[0]_DQS[3]
A9   B9   200m   NA
|DDR[1]_DQS[0]   DDR[1]_DQS[0]N
F34   E35   200m   NA
|DDR[1]_DQS[2]   DDR[1]_DQS[2]N
B30   A30   200m   NA
|DDR[1]_DQS[1]   DDR[1]_DQS[1]N
B34   A34   200m   NA
|DDR[0]_DQS[0]   DDR[0]_DQS[0]N
F4   E3   200m   NA
|   Usage I/O#1.5V###BSHTLTCSCDDVGPBFZ.*
|   Base model BSHTLTCSCDDVGPBFZ
[Model Selector] Selector_1
Model_304 3-STATE,1.5V,SLOWEST, 11MA,IND,10%
Model_305 3-STATE,1.5V,FAST, 8MA,IND,10%
Model_306 3-STATE,1.5V,FASTEST, 6MA,IND,10%
Model_307 3-STATE,1.5V,SLOW, 8MA,IND,10%
Model_308 3-STATE,1.5V,FASTEST, 10MA,IND,10%
Model_309 3-STATE,1.5V,FASTEST, 9MA,IND,10%
Model_310 3-STATE,1.5V,FAST, 10MA,IND,10%
Model_311 3-STATE,1.5V,SLOWEST, 6MA,IND,10%
Model_312 3-STATE,1.5V,FAST, 7MA,IND,10%
Model_313 3-STATE,1.5V,SLOW, 10MA,IND,10%
Model_314 3-STATE,1.5V,SLOW, 7MA,IND,10%
Model_315 3-STATE,1.5V,FAST, 11MA,IND,10%
Model_316 3-STATE,1.5V,SLOWEST, 7MA,IND,10%
Model_317 3-STATE,1.5V,SLOW, 11MA,IND,10%
Model_318 3-STATE,1.5V,FASTEST8MA,IND,10%
Model_319 3-STATE,1.5V,FAST, 6MA,IND,10%
Model_320 3-STATE,1.5V,FASTEST, 5MA,IND,10%
Model_321 3-STATE,1.5V,FAST, 5MA,IND,10%
Model_322 3-STATE,1.5V,SLOW, 6MA,IND,10%
Model_323 3-STATE,1.5V,SLOWEST, 8MA,IND,10%
Model_324 3-STATE,1.5V,SLOW, 5MA,IND,10%
Model_325 3-STATE,1.5V,FASTEST, 7MA,IND,10%
Model_326 3-STATE,1.5V,FAST, 9MA,IND,10%
Model_327 3-STATE,1.5V,SLOWEST, 5MA,IND,10%
Model_328 3-STATE,1.5V,SLOW, 9MA,IND,10%
Model_329 3-STATE,1.5V,FASTEST, 11MA,IND,10%
Model_330 3-STATE,1.5V,SLOWEST, 10MA,IND,10%
Model_331 3-STATE,1.5V,SLOWEST, 9MA,IND,10%
Model_360 3-STATE,1.5V,SLOWEST, 11MA,IND,5%
Model_361 3-STATE,1.5V,FAST, 8MA,IND,5%
Model_362 3-STATE,1.5V,FASTEST, 6MA,IND,5%
Model_363 3-STATE,1.5V,SLOW, 8MA,IND,5%
Model_364 3-STATE,1.5V,FASTEST, 10MA,IND,5%
Model_365 3-STATE,1.5V,FASTEST, 9MA,IND,5%
Model_366 3-STATE,1.5V,FAST, 10MA,IND,5%
Model_367 3-STATE,1.5V,SLOWEST, 6MA,IND,5%
Model_368 3-STATE,1.5V,FAST, 7MA,IND,5%
Model_369 3-STATE,1.5V,SLOW, 10MA,IND,5%
Model_370 3-STATE,1.5V,SLOW, 7MA,IND,5%
Model_371 3-STATE,1.5V,FAST, 11MA,IND,5%
Model_372 3-STATE,1.5V,SLOWEST, 7MA,IND,5%
Model_373 3-STATE,1.5V,SLOW, 11MA,IND,5%
Model_374 3-STATE,1.5V,FASTEST, 8MA,IND,5%
Model_375 3-STATE,1.5V,FAST, 6MA,IND,5%
Model_376 3-STATE,1.5V,FASTEST, 5MA,IND,5%
Model_377 3-STATE,1.5V,FAST, 5MA,IND,5%
Model_378 3-STATE,1.5V,SLOW, 6MA,IND,5%
Model_379 3-STATE,1.5V,SLOWEST, 8MA,IND,5%
Model_380 3-STATE,1.5V,SLOW, 5MA,IND,5%
Model_381 3-STATE,1.5V,FASTEST, 7MA,IND,5%
Model_382 3-STATE,1.5V,FAST, 9MA,IND,5%
Model_383 3-STATE,1.5V,SLOWEST, 5MA,IND,5%
Model_384 3-STATE,1.5V,SLOW, 9MA,IND,5%
Model_385 3-STATE,1.5V,FASTEST, 11MA,IND,5%
Model_386 3-STATE,1.5V,SLOWEST, 10MA,IND,5%
Model_387 3-STATE,1.5V,SLOWEST, 9MA,IND,5%
Model_416 3-STATE,1.5V,SLOWEST, 11MA,IND,10%
Model_417 3-STATE,1.5V,FAST, 8MA,IND,10%
Model_418 3-STATE,1.5V,FASTEST, 6MA,IND,10%
Model_419 3-STATE,1.5V,SLOW, 8MA,IND,10%
Model_420 3-STATE,1.5V,FASTEST, 10MA,IND,10%
Model_421 3-STATE,1.5V,FASTEST, 9MA,IND,10%
Model_422 3-STATE,1.5V,FAST, 10MA,IND,10%
Model_423 3-STATE,1.5V,SLOWEST, 6MA,IND,10%
Model_424 3-STATE,1.5V,FAST, 7MA,IND,10%
Model_425 3-STATE,1.5V,SLOW, 10MA,IND,10%
Model_426 3-STATE,1.5V,SLOW, 7MA,IND,10%
Model_427 3-STATE,1.5V,FAST, 11MA,IND,10%
Model_428 3-STATE,1.5V,SLOWEST, 7MA,IND,10%
Model_429 3-STATE,1.5V,SLOW, 11MA,IND,10%
Model_430 3-STATE,1.5V,FASTEST, 8MA,IND,10%
Model_431 3-STATE,1.5V,FAST, 6MA,IND,10%
Model_432 3-STATE,1.5V,FASTEST, 5MA,IND,10%
Model_433 3-STATE,1.5V,FAST, 5MA,IND,10%
Model_434 3-STATE,1.5V,SLOW, 6MA,IND,10%
Model_435 3-STATE,1.5V,SLOWEST, 8MA,IND,10%
Model_436 3-STATE,1.5V,SLOW, 5MA,IND,10%
Model_437 3-STATE,1.5V,FASTEST, 7MA,IND,10%
Model_438 3-STATE,1.5V,FAST, 9MA,IND,10%
Model_439 3-STATE,1.5V,SLOWEST, 5MA,IND,10%
Model_440 3-STATE,1.5V,SLOW, 9MA,IND,10%
Model_441 3-STATE,1.5V,FASTEST, 11MA,IND,10%
Model_442 3-STATE,1.5V,SLOWEST, 10MA,IND,10%
Model_443 3-STATE,1.5V,SLOWEST, 9MA,IND,10%
Model_472 3-STATE,1.5V,SLOWEST, 11MA,IND,5%
Model_473 3-STATE,1.5V,FAST, 8MA,IND,5%
Model_474 3-STATE,1.5V,FASTEST, 6MA,IND,5%
Model_475 3-STATE,1.5V,SLOW, 8MA,IND,5%
Model_476 3-STATE,1.5V,FASTEST, 10MA,IND,5%
Model_477 3-STATE,1.5V,FASTEST, 9MA,IND,5%
Model_478 3-STATE,1.5V,FAST, 10MA,IND,5%
Model_479 3-STATE,1.5V,SLOWEST, 6MA,IND,5%
Model_480 3-STATE,1.5V,FAST, 7MA,IND,5%
Model_481 3-STATE,1.5V,SLOW, 10MA,IND,5%
Model_482 3-STATE,1.5V,SLOW, 7MA,IND,5%
Model_483 3-STATE,1.5V,FAST, 11MA,IND,5%
Model_484 3-STATE,1.5V,SLOWEST, 7MA,IND,5%
Model_485 3-STATE,1.5V,SLOW, 11MA,IND,5%
Model_486 3-STATE,1.5V,FASTEST, 8MA,IND,5%
Model_487 3-STATE,1.5V,FAST, 6MA,IND,5%
Model_488 3-STATE,1.5V,FASTEST, 5MA,IND,5%
Model_489 3-STATE,1.5V,FAST, 5MA,IND,5%
Model_490 3-STATE,1.5V,SLOW, 6MA,IND,5%
Model_491 3-STATE,1.5V,SLOWEST, 8MA,IND,5%
Model_492 3-STATE,1.5V,SLOW, 5MA,IND,5%
Model_493 3-STATE,1.5V,FASTEST, 7MA,IND,5%
Model_494 3-STATE,1.5V,FAST, 9MA,IND,5%
Model_495 3-STATE,1.5V,SLOWEST, 5MA,IND,5%
Model_496 3-STATE,1.5V,SLOW, 9MA,IND,5%
Model_497 3-STATE,1.5V,FASTEST, 11MA,IND,5%
Model_498 3-STATE,1.5V,SLOWEST, 10MA,IND,5%
Model_499 3-STATE,1.5V,SLOWEST, 9MA,IND,5%
Model_663 INPUT,1.5V,DIFF_HALFTERM, 9MA,IND,10%
Model_664 INPUT,1.5V,DIFF_HALFTERM, 5MA,IND,10%
Model_665 INPUT,1.5V,DIFF_FULLTERM, 11MA,IND,10%
Model_666 INPUT,1.5V,DIFF_FULLTERM, 7MA,IND,10%
Model_667 INPUT,1.5V,DIFF_HALFTERM, 7MA,IND,10%
Model_668 INPUT,1.5V,DIFF_HALFTERM, 11MA,IND,10%
Model_669 INPUT,1.5V,NOTERM, Pull-up,IND,10%
Model_670 INPUT,1.5V,NOTERM, Pull-up/down off,IND,10%
Model_671 INPUT,1.5V,NOTERM, Pull-down,IND,10%
Model_672 INPUT,1.5V,DIFF_FULLTERM, 8MA,IND,10%
Model_673 INPUT,1.5V,DIFF_HALFTERM, 8MA,IND,10%
Model_674 INPUT,1.5V,DIFF_FULLTERM, 10MA,IND,10%
Model_675 INPUT,1.5V,DIFF_FULLTERM, 6MA,IND,10%
Model_676 INPUT,1.5V,DIFF_FULLTERM, 9MA,IND,10%
Model_677 INPUT,1.5V,DIFF_HALFTERM, 10MA,IND,10%
Model_678 INPUT,1.5V,DIFF_FULLTERM, 5MA,IND,10%
Model_679 INPUT,1.5V,DIFF_HALFTERM, 6MA,IND,10%
|   Usage I/O#3.3V#PD/PI/PU##BC3340DGHYPBFBP18.PAD
|   Base model BC3340DGHYPBFBP18
[Model Selector] Selector_2
Model_714 INPUT,3.3V,Pull-down
Model_715 INPUT,3.3V,Pull-up
Model_716 I/O,3.3V,Pull-up/down off
|   Usage INPUT#3.3V#PD/PI/PU##IQ33GHYPBFBP18.PAD
|   Base model IQ33GHYPBFBP18
[Model Selector] Selector_3
Model_717 INPUT,3.3V,Pull-down
Model_718 INPUT,3.3V,Pull-up
Model_719 INPUT,3.3V,Pull-up/down off
|   Usage I/O#1.5V###BSHTLTCSCDVGPBFZ.PAD
|   Base model BSHTLTCSCDVGPBFZ
[Model Selector] Selector_4
Model_100 3-STATE,1.5V,FASTEST, 8MA,IND,5%
Model_101 3-STATE,1.5V,FAST, 6MA,IND,5%
Model_102 3-STATE,1.5V,FASTEST, 5MA,IND,5%
Model_103 3-STATE,1.5V,FAST, 5MA,IND,5%
Model_104 3-STATE,1.5V,SLOW, 6MA,IND,5%
Model_105 3-STATE,1.5V,SLOWEST, 8MA,IND,5%
Model_106 3-STATE,1.5V,SLOW, 5MA,IND,5%
Model_107 3-STATE,1.5V,FASTEST, 7MA,IND,5%
Model_108 3-STATE,1.5V,FAST, 9MA,IND,5%
Model_109 3-STATE,1.5V,SLOWEST, 5MA,IND,5%
Model_110 3-STATE,1.5V,SLOW, 9MA,IND,5%
Model_111 3-STATE,1.5V,FASTEST, 11MA,IND,5%
Model_112 3-STATE,1.5V,SLOWEST, 10MA,IND,5%
Model_113 3-STATE,1.5V,SLOWEST, 9MA,IND,5%
Model_221 INPUT,1.5V,HALFTERM, 9MA,IND,10%
Model_222 INPUT,1.5V,HALFTERM, 5MA,IND,10%
Model_223 INPUT,1.5V,FULLTERM, 11MA,IND,10%
Model_224 INPUT,1.5V,FULLTERM, 7MA,IND,10%
Model_225 INPUT,1.5V,HALFTERM, 7MA,IND,10%
Model_226 INPUT,1.5V,HALFTERM, 11MA,IND,10%
Model_227 INPUT,1.5V,NOTERM,IND,10%
Model_228 INPUT,1.5V,NOTERM,IND,10%
Model_229 INPUT,1.5V,NOTERM,IND,10%
Model_230 INPUT,1.5V,FULLTERM, 8MA,IND,10%
Model_231 INPUT,1.5V,HALFTERM, 8MA,IND,10%
Model_232 INPUT,1.5V,FULLTERM, 10MA,IND,10%
Model_233 INPUT,1.5V,FULLTERM, 6MA,IND,10%
Model_234 INPUT,1.5V,FULLTERM, 9MA,IND,10%
Model_235 INPUT,1.5V,HALFTERM, 10MA,IND,10%
Model_236 INPUT,1.5V,FULLTERM, 5MA,IND,10%
Model_237 INPUT,1.5V,HALFTERM, 6MA,IND,10%
Model_30 3-STATE,1.5V,SLOWEST, 11MA,IND,10%
Model_31 3-STATE,1.5V,FAST, 8MA,IND,10%
Model_32 3-STATE,1.5V,FASTEST, 6MA,IND,10%
Model_33 3-STATE,1.5V,SLOW, 8MA,IND,10%
Model_34 3-STATE,1.5V,FASTEST, 10MA,IND,10%
Model_35 3-STATE,1.5V,FASTEST, 9MA,IND,10%
Model_36 3-STATE,1.5V,FAST, 10MA,IND,10%
Model_37 3-STATE,1.5V,SLOWEST, 6MA,IND,10%
Model_38 3-STATE,1.5V,FAST, 7MA,IND,10%
Model_39 3-STATE,1.5V,SLOW, 10MA,IND,10%
Model_40 3-STATE,1.5V,SLOW, 7MA,IND,10%
Model_41 3-STATE,1.5V,FAST, 11MA,IND,10%
Model_42 3-STATE,1.5V,SLOWEST, 7MA,IND,10%
Model_43 3-STATE,1.5V,SLOW, 11MA,IND,10%
Model_44 3-STATE,1.5V,FASTEST, 8MA,IND,10%
Model_45 3-STATE,1.5V,FAST, 6MA,IND,10%
Model_46 3-STATE,1.5V,FASTEST, 5MA,IND,10%
Model_47 3-STATE,1.5V,FAST, 5MA,IND,10%
Model_48 3-STATE,1.5V,SLOW, 6MA,IND,10%
Model_49 3-STATE,1.5V,SLOWEST, 8MA,IND,10%
Model_50 3-STATE,1.5V,SLOW, 5MA,IND,10%
Model_51 3-STATE,1.5V,FASTEST, 7MA,IND,10%
Model_52 3-STATE,1.5V,FAST, 9MA,IND,10%
Model_53 3-STATE,1.5V,SLOWEST, 5MA,IND,10%
Model_54 3-STATE,1.5V,SLOW, 9MA,IND,10%
Model_55 3-STATE,1.5V,FASTEST, 11MA,IND,10%
Model_56 3-STATE,1.5V,SLOWEST, 10MA,IND,10%
Model_57 3-STATE,1.5V,SLOWEST, 9MA,IND,10%
Model_86 3-STATE,1.5V,SLOWEST, 11MA,IND,5%
Model_87 3-STATE,1.5V,FAST, 8MA,IND,5%
Model_88 3-STATE,1.5V,FASTEST, 6MA,IND,5%
Model_89 3-STATE,1.5V,SLOW, 8MA,IND,5%
Model_90 3-STATE,1.5V,FASTEST, 10MA,IND,5%
Model_91 3-STATE,1.5V,FASTEST, 9MA,IND,5%
Model_92 3-STATE,1.5V,FAST, 10MA,IND,5%
Model_93 3-STATE,1.5V,SLOWEST, 6MA,IND,5%
Model_94 3-STATE,1.5V,FAST, 7MA,IND,5%
Model_95 3-STATE,1.5V,SLOW, 10MA,IND,5%
Model_96 3-STATE,1.5V,SLOW, 7MA,IND,5%
Model_97 3-STATE,1.5V,FAST, 11MA,IND,5%
Model_98 3-STATE,1.5V,SLOWEST, 7MA,IND,5%
Model_99 3-STATE,1.5V,SLOW, 11MA,IND,5%
|   Usage I/O#3.3V#PD/PI/PU##BC3340CGHYPBFBP18.PAD
|   Base model BC3340CGHYPBFBP18
[Model Selector] Selector_5
Model_272 INPUT,3.3V,Pull-down
Model_273 INPUT,3.3V,Pull-up
Model_274 I/O,3.3V,Pull-up/down off
|   Usage OUTPUT#1.5V###BSHTLTCSCDVGPBFZ.PAD
|   Base model BSHTLTCSCDVGPBFZ
[Model Selector] Selector_6
Model_100 3-STATE,1.5V,FASTEST, 8MA,IND,5%
Model_101 3-STATE,1.5V,FAST, 6MA,IND,5%
Model_102 3-STATE,1.5V,FASTEST, 5MA,IND,5%
Model_103 3-STATE,1.5V,FAST, 5MA,IND,5%
Model_104 3-STATE,1.5V,SLOW, 6MA,IND,5%
Model_105 3-STATE,1.5V,SLOWEST, 8MA,IND,5%
Model_106 3-STATE,1.5V,SLOW, 5MA,IND,5%
Model_107 3-STATE,1.5V,FASTEST, 7MA,IND,5%
Model_108 3-STATE,1.5V,FAST, 9MA,IND,5%
Model_109 3-STATE,1.5V,SLOWEST, 5MA,IND,5%
Model_110 3-STATE,1.5V,SLOW, 9MA,IND,5%
Model_111 3-STATE,1.5V,FASTEST, 11MA,IND,5%
Model_112 3-STATE,1.5V,SLOWEST, 10MA,IND,5%
Model_113 3-STATE,1.5V,SLOWEST, 9MA,IND,5%
Model_30 3-STATE,1.5V,SLOWEST, 11MA,IND,10%
Model_31 3-STATE,1.5V,FAST, 8MA,IND,10%
Model_32 3-STATE,1.5V,FASTEST, 6MA,IND,10%
Model_33 3-STATE,1.5V,SLOW, 8MA,IND,10%
Model_34 3-STATE,1.5V,FASTEST, 10MA,IND,10%
Model_35 3-STATE,1.5V,FASTEST, 9MA,IND,10%
Model_36 3-STATE,1.5V,FAST, 10MA,IND,10%
Model_37 3-STATE,1.5V,SLOWEST, 6MA,IND,10%
Model_38 3-STATE,1.5V,FAST, 7MA,IND,10%
Model_39 3-STATE,1.5V,SLOW, 10MA,IND,10%
Model_40 3-STATE,1.5V,SLOW, 7MA,IND,10%
Model_41 3-STATE,1.5V,FAST, 11MA,IND,10%
Model_42 3-STATE,1.5V,SLOWEST, 7MA,IND,10%
Model_43 3-STATE,1.5V,SLOW, 11MA,IND,10%
Model_44 3-STATE,1.5V,FASTEST, 8MA,IND,10%
Model_45 3-STATE,1.5V,FAST, 6MA,IND,10%
Model_46 3-STATE,1.5V,FASTEST, 5MA,IND,10%
Model_47 3-STATE,1.5V,FAST, 5MA,IND,10%
Model_48 3-STATE,1.5V,SLOW, 6MA,IND,10%
Model_49 3-STATE,1.5V,SLOWEST, 8MA,IND,10%
Model_50 3-STATE,1.5V,SLOW, 5MA,IND,10%
Model_51 3-STATE,1.5V,FASTEST, 7MA,IND,10%
Model_52 3-STATE,1.5V,FAST, 9MA,IND,10%
Model_53 3-STATE,1.5V,SLOWEST, 5MA,IND,10%
Model_54 3-STATE,1.5V,SLOW, 9MA,IND,10%
Model_55 3-STATE,1.5V,FASTEST, 11MA,IND,10%
Model_56 3-STATE,1.5V,SLOWEST, 10MA,IND,10%
Model_57 3-STATE,1.5V,SLOWEST, 9MA,IND,10%
Model_86 3-STATE,1.5V,SLOWEST, 11MA,IND,5%
Model_87 3-STATE,1.5V,FAST, 8MA,IND,5%
Model_88 3-STATE,1.5V,FASTEST, 6MA,IND,5%
Model_89 3-STATE,1.5V,SLOW, 8MA,IND,5%
Model_90 3-STATE,1.5V,FASTEST, 10MA,IND,5%
Model_91 3-STATE,1.5V,FASTEST, 9MA,IND,5%
Model_92 3-STATE,1.5V,FAST, 10MA,IND,5%
Model_93 3-STATE,1.5V,SLOWEST, 6MA,IND,5%
Model_94 3-STATE,1.5V,FAST, 7MA,IND,5%
Model_95 3-STATE,1.5V,SLOW, 10MA,IND,5%
Model_96 3-STATE,1.5V,SLOW, 7MA,IND,5%
Model_97 3-STATE,1.5V,FAST, 11MA,IND,5%
Model_98 3-STATE,1.5V,SLOWEST, 7MA,IND,5%
Model_99 3-STATE,1.5V,SLOW, 11MA,IND,5%
| Models and submodels in the file (213): Model_1 (Input), Model_30 (3-state), Model_31 (3-state), Model_32 (3-state), Model_33 (3-state), Model_34 (3-state), Model_35 (3-state), Model_36 (3-state), Model_37 (3-state), Model_38 (3-state), Model_39 (3-state), Model_40 (3-state), Model_41 (3-state), Model_42 (3-state), Model_43 (3-state), Model_44 (3-state), Model_45 (3-state), Model_46 (3-state), Model_47 (3-state), Model_48 (3-state), Model_49 (3-state), Model_50 (3-state), Model_51 (3-state), Model_52 (3-state), Model_53 (3-state), Model_54 (3-state), Model_55 (3-state), Model_56 (3-state), Model_57 (3-state), Model_86 (3-state), Model_87 (3-state), Model_88 (3-state), Model_89 (3-state), Model_90 (3-state), Model_91 (3-state), Model_92 (3-state), Model_93 (3-state), Model_94 (3-state), Model_95 (3-state), Model_96 (3-state), Model_97 (3-state), Model_98 (3-state), Model_99 (3-state), Model_100 (3-state), Model_101 (3-state), Model_102 (3-state), Model_103 (3-state), Model_104 (3-state), Model_105 (3-state), Model_106 (3-state), Model_107 (3-state), Model_108 (3-state), Model_109 (3-state), Model_110 (3-state), Model_111 (3-state), Model_112 (3-state), Model_113 (3-state), Model_221 (Input), Model_222 (Input), Model_223 (Input), Model_224 (Input), Model_225 (Input), Model_226 (Input), Model_227 (Input), Model_228 (Input), Model_229 (Input), Model_230 (Input), Model_231 (Input), Model_232 (Input), Model_233 (Input), Model_234 (Input), Model_235 (Input), Model_236 (Input), Model_237 (Input), Model_272 (Input), Model_273 (Input), Model_274 (I/O), Model_275 (I/O_open_drain), Model_304 (3-state), Model_305 (3-state)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
